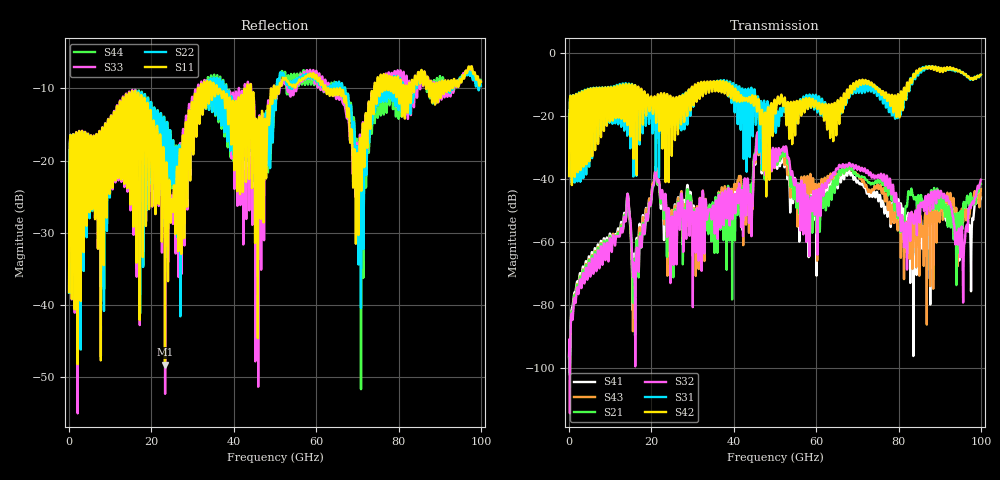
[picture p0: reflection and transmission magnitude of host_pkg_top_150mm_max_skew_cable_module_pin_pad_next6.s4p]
# Hz S RI R 50
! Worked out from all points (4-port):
!   10000 points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, 10 MHz to 100 GHz, reference 50 ohm
!   strongest paths, dB at 10 MHz, 25.01 GHz, 50.01 GHz, 75.01 GHz, 100 GHz:
!     S42: -39.1, -23.6, -16.0, -11.7, -6.9
!     S31: -39.0, -20.9, -22.3, -12.0, -6.9
!     S32: -96.0, -52.0, -35.1, -38.7, -40.2
!     S21: -96.4, -52.3, -34.5, -40.4, -41.5
!     S43: -96.4, -49.8, -35.4, -42.3, -43.1
!     S41: -96.8, -49.9, -35.1, -46.3, -45.9
!   lowest |S11| = -48.3 dB at 23.29 GHz (marker M1), VSWR 1.01, Z = 49.7 + j0.255 ohm
!   |S11| at or under -10 dB: start of sweep to 31.27 GHz; 35.95 GHz to 42.6 GHz (6.648 GHz wide, 16.9 % of centre); 65.82 GHz to 74.11 GHz (8.291 GHz wide, 11.8 % of centre)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
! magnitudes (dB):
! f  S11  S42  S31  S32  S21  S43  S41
! 10 MHz  -38.2  -39.1  -39.0  -96.0  -96.4  -96.4  -96.8
! 23.29 GHz  -48.3  -16.9  -20.8  -45.2  -45.7  -47.6  -47.7
! 44.11 GHz  -9.7  -15.9  -12.3  -47.0  -44.8  -50.6  -46.5
! 46.1 GHz  -14.2  -15.1  -25.6  -30.7  -30.0  -32.1  -31.9
! 60.47 GHz  -9.0  -17.1  -15.9  -47.8  -48.1  -43.1  -45.8
! 95.41 GHz  -8.7  -6.1  -6.3  -55.9  -56.1  -49.4  -55.7
! 100 GHz  -9.1  -6.9  -6.9  -40.2  -41.5  -43.1  -45.9
